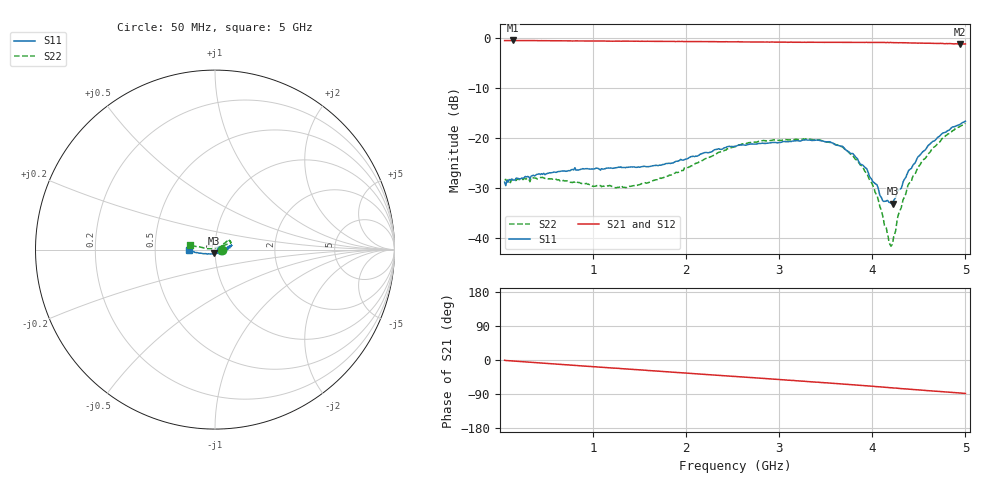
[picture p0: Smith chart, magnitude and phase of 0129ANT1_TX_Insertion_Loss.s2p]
! MASWSS0129 de-embedded Sparameters using port extention method. ANT1 to TX Insertion Loss using 3 volt control
! Board loss is removed and phase length of connector and line length of board are dialed out
! 100pF blocking capacitor
! Sample board 1000013136
#	Hz	S	DB	R	50
!	Freq	S11	S21	S12	S22
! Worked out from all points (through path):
!   401 points, 50 MHz to 5 GHz, reference 50 ohm
!   highest |S21| = -0.51 dB at 137 MHz (marker M1); lowest = -1.2 dB at 4.94 GHz (marker M2)
!   group delay of S21, straight-line fit = 48.4 ps
!   lowest |S11| = -33.1 dB at 4.22 GHz (marker M3), VSWR 1.05, Z = 49.4 - j2.13 ohm
!   |S11| at or under -10 dB: start of sweep to end of sweep
!   |S22| runs from -41.6 to -17.0 dB; largest |S21 - S12| = 0.0087
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5e7  -28.83 0.1  -0.53 -0.7  -0.49 -1.2  -28.34 -0.2
1.37e8  -28.38 0.6  -0.51 -2.4  -0.50 -2.6  -28.26 1.1
4.58e8  -27.26 2.5  -0.55 -8.3  -0.55 -8.3  -27.86 6.5
8.79e8  -26.19 -7.6  -0.61 -15.6  -0.58 -15.6  -29.08 1.2
1.35e9  -25.92 -6.4  -0.65 -23.5  -0.64 -23.5  -29.90 12.3
1.7e9  -25.52 2.3  -0.68 -29.4  -0.69 -29.4  -28.33 27.7
2.53e9  -21.64 12.6  -0.79 -43.6  -0.79 -43.6  -21.74 35.1
2.82e9  -21.03 13.4  -0.82 -48.5  -0.83 -48.6  -20.55 33.5
3.35e9  -20.49 14.1  -0.87 -57.8  -0.88 -57.8  -20.32 23.8
3.68e9  -21.67 6.8  -0.89 -63.2  -0.89 -63.4  -21.77 22.6
3.89e9  -25.32 -8.2  -0.89 -67.1  -0.90 -67.3  -25.58 26.3
4.05e9  -29.34 -31.7  -0.91 -70.3  -0.89 -70.3  -31.43 37.1
4.11e9  -32.47 -52.2  -0.93 -71.5  -0.92 -71.5  -35.44 47.6
4.18e9  -32.84 -83.0  -0.92 -72.9  -0.93 -73.0  -40.87 89.4
4.22e9  -33.11 -103.5  -0.94 -73.6  -0.94 -73.8  -40.86 123.7
4.25e9  -31.90 -116.6  -0.94 -74.0  -0.96 -74.3  -38.60 142.2
4.29e9  -30.24 -129.1  -0.96 -75.0  -0.95 -75.1  -34.77 161.5
4.34e9  -28.38 -141.1  -0.98 -76.1  -0.97 -76.2  -31.98 166.8
4.49e9  -23.77 -159.5  -1.03 -78.8  -1.03 -79.0  -25.83 171.7
4.76e9  -19.00 -171.8  -1.12 -83.9  -1.14 -84.3  -19.85 170.0
4.94e9  -17.29 -177.3  -1.21 -87.0  -1.19 -87.4  -17.69 170.9
5e9  -16.64 -178.4  -1.21 -88.3  -1.22 -88.5  -17.04 170.6
